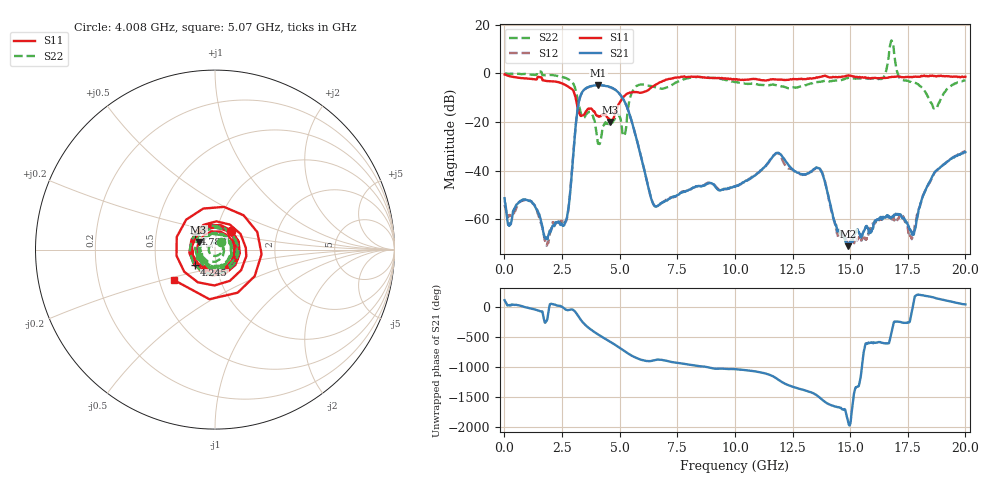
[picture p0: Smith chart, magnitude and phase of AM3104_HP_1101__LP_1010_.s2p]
!Created with skrf (http://scikit-rf.org).
# Hz S RI R 50.0
!freq ReS11 ImS11 ReS21 ImS21 ReS12 ImS12 ReS22 ImS22
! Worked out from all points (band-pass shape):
!   1601 points, 10 MHz to 20 GHz, reference 50 ohm
!   highest |S21| = -4.77 dB at 4.083 GHz (marker M1); lowest = -71.2 dB at 14.93 GHz (marker M2)
!   |S21| within 3 dB of the highest: 3.371 GHz to 4.934 GHz (1.563 GHz wide, 37.6 % of centre)
!   lowest |S11| = -20.0 dB at 4.595 GHz (marker M3), VSWR 1.22, Z = 41.5 + j3.51 ohm
!   |S11| at or under -10 dB: 3.089 GHz to 5.139 GHz (2.05 GHz wide, 49.8 % of centre)
!   |S22| runs from -29.1 to 13.6 dB; largest |S21 - S12| = 0.048
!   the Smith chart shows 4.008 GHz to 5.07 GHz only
!   S11 on the Smith chart (normalised r, x): 4.008 GHz: 1.17, +0.25; 4.245 GHz: 0.79, -0.14; 4.783 GHz: 0.78, +0.14; 5.07 GHz: 0.60, -0.22
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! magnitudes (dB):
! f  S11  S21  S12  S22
! 10 MHz  -0.4  -51.4  -54.1  0.0
! 222.4 MHz  -1.1  -62.7  -58.6  -0.1
! 1.172 GHz  -2.2  -52.8  -52.8  -0.5
! 1.834 GHz  -3.1  -68.2  -71.0  -0.7
! 2.609 GHz  -4.6  -62.2  -61.3  -1.7
! 3.346 GHz  -17.4  -8.2  -8.3  -17.1
! 4.008 GHz  -17.3  -4.8  -4.9  -25.4
! 4.083 GHz  -17.5  -4.8  -4.8  -28.7
! 4.245 GHz  -16.9  -4.9  -4.9  -23.4
! 4.595 GHz  -20.0  -5.6  -5.8  -21.2
! 4.783 GHz  -16.8  -6.5  -6.6  -18.8
! 5.07 GHz  -10.9  -9.3  -9.3  -20.2
! 5.695 GHz  -7.6  -25.6  -25.6  -5.5
! 6.682 GHz  -4.0  -54.4  -54.4  -6.0
! 10.01 GHz  -2.5  -46.8  -46.6  -3.6
! 11.83 GHz  -2.5  -32.8  -32.9  -5.0
! 13.34 GHz  -2.1  -40.3  -40.3  -4.1
! 14.93 GHz  -0.8  -71.2  -69.0  -1.7
! 16.68 GHz  -1.6  -59.2  -59.3  7.2
! 17.69 GHz  -1.5  -66.4  -67.8  -3.7
! 18.68 GHz  -1.0  -40.6  -40.7  -14.2
! 20 GHz  -1.3  -32.4  -32.0  -2.8
